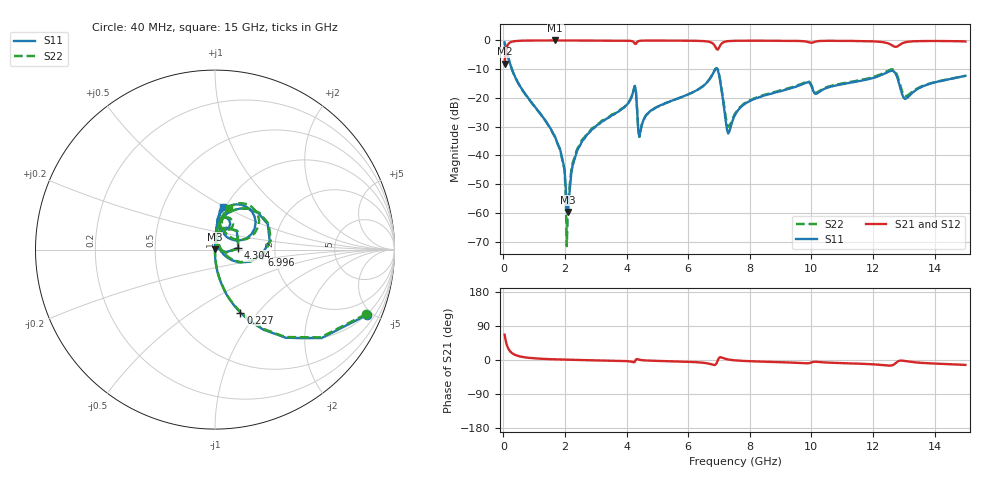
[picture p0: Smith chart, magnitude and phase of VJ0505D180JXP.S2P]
! VJ0505D180JXP
! MLCC placed on 25 mil thick microstrip substrate in series configuraton.
! DATE 06/29/2018  09:04
! CORRECTED  DATA
# GHz  S  MA  R  50.00
!  FREQ  S11M  S11A  S21M  S21A  S12M  S12A  S22M  S22A
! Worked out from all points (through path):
!   401 points, 40 MHz to 15 GHz, reference 50 ohm
!   highest |S21| = -0.01 dB at 1.686 GHz (marker M1); lowest = -8.1 dB at 40 MHz (marker M2)
!   group delay of S21, straight-line fit = 3.49 ps
!   lowest |S11| = -59.7 dB at 2.097 GHz (marker M3), VSWR 1.00, Z = 49.9 + j0.0818 ohm
!   |S11| at or under -10 dB: 276.6 MHz to 6.886 GHz (6.609 GHz wide, 185 % of centre); 6.942 GHz to end of sweep
!   |S22| runs from -71.6 to -0.8 dB; largest |S21 - S12| = 0.0024
!   S11 on the Smith chart (normalised r, x): 40 MHz: 0.96, -4.68; 227 MHz: 1.00, -0.82; 4.304 GHz: 1.30, +0.03; 6.996 GHz: 1.70, -0.11; 15 GHz: 0.97, +0.49
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0.04  0.9223 -23.2  0.3947 66.8  0.395 66.7  0.9141 -23.2
0.227  0.3781 -68.1  0.9261 22.2  0.9267 22.3  0.3747 -67.9
0.6758  0.1241 -83.7  0.9922 7.3  0.9928 7.4  0.1229 -83.6
1.6856  0.02059 -90.5  0.9992 1.7  0.999 1.8  0.02049 -90.5
1.91  0.008736 -93.7  0.9971 1.2  0.9987 1.2  0.008405 -92.6
2.0222  0.002883 -102.6  0.9984 0.8  0.9985 0.9  0.002122 -85.5
2.097  0.001034 127.6  0.998 0.7  0.9984 0.8  0.001393 84.3
2.284  0.007712 93.3  0.9973 0.4  0.9978 0.4  0.008361 87.5
2.5458  0.0173 90.8  0.997 -0.1  0.9973 -0.0  0.01833 86.3
4.2288  0.1372 63.3  0.9395 -5.9  0.9398 -5.8  0.1381 61.6
4.3036  0.1301 4.5  0.8693 1.2  0.8696 1.2  0.1306 2.6
4.4532  0.02691 69.7  0.9877 0.1  0.9881 0.2  0.02734 67.5
5.0516  0.07213 87.7  0.9943 -2.4  0.9948 -2.4  0.07162 85.7
6.8094  0.2683 58.5  0.8767 -12.8  0.8776 -12.7  0.2717 57.6
6.9964  0.2619 -6.9  0.7378 5.1  0.7384 5.1  0.2694 -6.2
7.2956  0.02403 21.9  0.9721 1.5  0.9725 1.5  0.03145 17.7
7.52  0.05083 81.0  0.9858 -0.9  0.9865 -0.9  0.05322 73.2
8.2306  0.09935 86.2  0.9904 -3.9  0.9904 -3.8  0.1022 82.7
10.0258  0.1483 57.8  0.9154 -5.6  0.9164 -5.6  0.1557 52.4
12.5316  0.2899 59.3  0.8708 -14.8  0.8715 -14.8  0.3048 57.1
13.0552  0.09642 51.1  0.9313 -3.0  0.9325 -3.0  0.1083 46.0
15  0.2421 79.8  0.961 -13.0  0.9614 -13.0  0.2436 70.8
